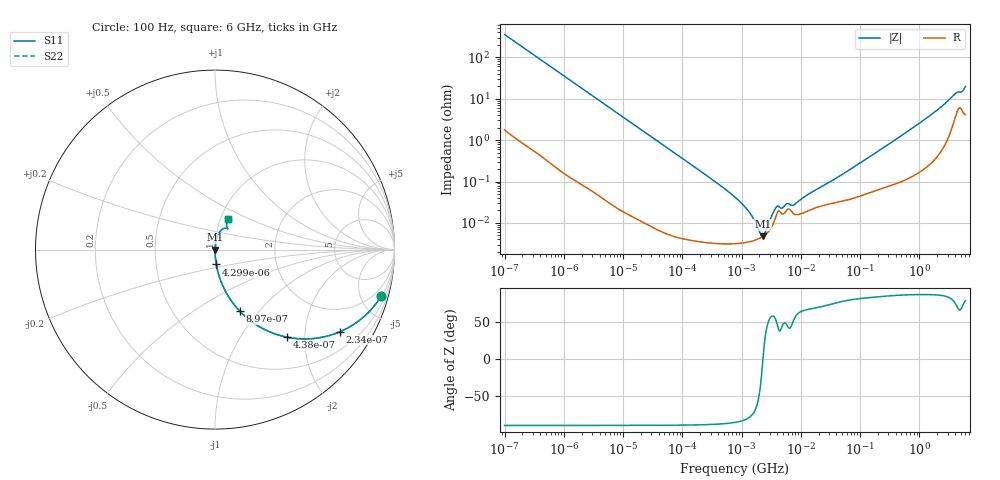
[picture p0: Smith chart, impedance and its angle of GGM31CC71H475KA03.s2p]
!Murata Part Number: GGM31CC71H475KA03
!These Parameters are Measured in Series Mode Connection
!Data Generated on Mar 13, 2026
!  o--ll--o
!Port1  Port2
!  o------o
!Operation Temp=25[degC], DC Bias Voltage=0[V]
!Freq. Start=100[Hz] Stop=6[GHz] 401[Steps]
# Hz S RI R 50
!Freq.(Hz) S11(Real) S11(Imag) S21(Real) S21(Imag) S12(Real) S12(Imag) S22(Real) S22(Imag)
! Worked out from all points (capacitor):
!   401 points, 100 Hz to 6 GHz, reference 50 ohm
!   read as one part in series: C = 4.47 uF near 109 Hz
!   lowest |Z| = 4.73 mohm at 2.269 MHz (marker M1)
!   series resonance near 2.297 MHz, so ESL is about 1.1 nH
!   S11 on the Smith chart (normalised r, x): 100 Hz: 1.04, -7.12; 234 Hz: 1.01, -3.05; 438 Hz: 1.01, -1.63; 897 Hz: 1.00, -0.80; 4.299 kHz: 1.00, -0.17; 6 GHz: 1.08, +0.39
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100  0.9257 -0.2598  0.0743 0.2598  0.0743 0.2598  0.9257 -0.2598
150  0.8488 -0.3559  0.1512 0.3559  0.1512 0.3559  0.8488 -0.3559
234  0.6979 -0.4568  0.3021 0.4568  0.3021 0.4568  0.6979 -0.4568
438  0.3998 -0.4875  0.6002 0.4875  0.6002 0.4875  0.3998 -0.4875
897  0.1385 -0.3432  0.8615 0.3432  0.8615 0.3432  0.1385 -0.3432
2008  0.0317 -0.1728  0.9683 0.1728  0.9683 0.1728  0.0317 -0.1728
4299  0.00735 -0.083  0.9926 0.083  0.9926 0.083  0.00735 -0.083
40335  0.000146 -0.00897  0.9999 0.00897  0.9999 0.00897  0.000146 -0.00897
774597  3.17e-05 -0.000418  1 0.000418  1 0.000418  3.17e-05 -0.000418
1212075  3.4e-05 -0.000219  1 0.000219  1 0.000219  3.4e-05 -0.000219
1734173  3.9e-05 -9.25e-05  1 9.25e-05  1 9.25e-05  3.9e-05 -9.25e-05
2268635  4.71e-05 -4e-06  1 4e-06  1 4e-06  4.71e-05 -4e-06
2837864  6.19e-05 7.39e-05  0.9999 -7.39e-05  0.9999 -7.39e-05  6.19e-05 7.39e-05
3882480  0.000159 0.000187  0.9998 -0.000187  0.9998 -0.000187  0.000159 0.000187
4856642  0.000164 0.000158  0.9998 -0.000158  0.9998 -0.000158  0.000164 0.000158
5809218  0.000205 0.000208  0.9998 -0.000208  0.9998 -0.000208  0.000205 0.000208
7599586  0.000168 0.000214  0.9998 -0.000214  0.9998 -0.000214  0.000168 0.000214
1.555665e7  0.000217 0.000519  0.9998 -0.000519  0.9998 -0.000519  0.000217 0.000519
3.124326e8  0.000846 0.00811  0.9992 -0.00811  0.9992 -0.00811  0.000846 0.00811
1.791126e9  0.00546 0.0464  0.9945 -0.0464  0.9945 -0.0464  0.00546 0.0464
4.009986e9  0.0473 0.1165  0.9527 -0.1165  0.9527 -0.1165  0.0473 0.1165
6e9  0.072 0.1727  0.928 -0.1727  0.928 -0.1727  0.072 0.1727
